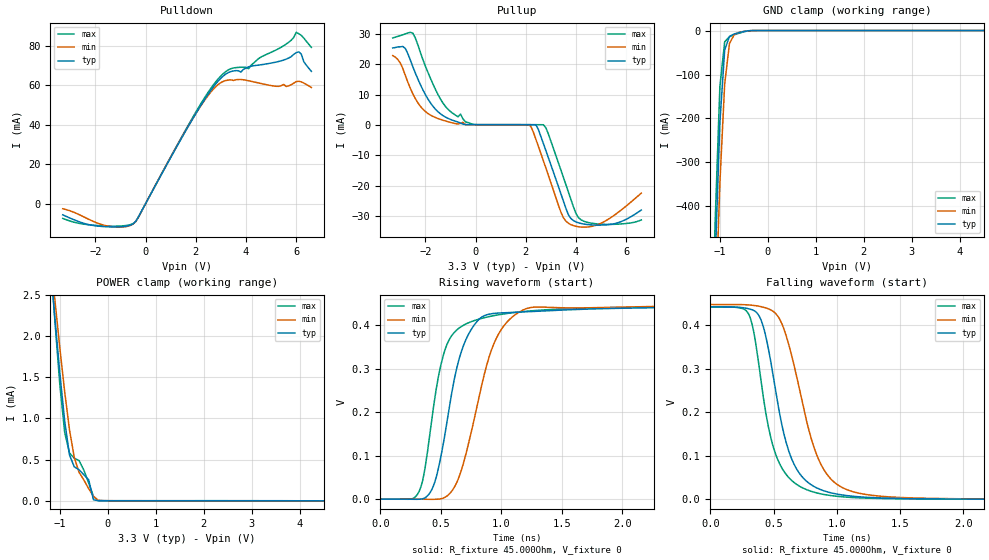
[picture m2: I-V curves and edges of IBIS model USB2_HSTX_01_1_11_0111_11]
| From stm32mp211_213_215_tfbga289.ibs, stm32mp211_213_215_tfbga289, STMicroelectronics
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[Model] USB2_HSTX_01_1_11_0111_11
Model_type   Output
Polarity   Non-Inverting
Enable   Active-High
C_comp   8.036pF   7.631pF   8.569pF
Vmeas = 200.000mV
Vref = 200.000mV
Rref = 45Ohms
Cref = 0pF
[Model Spec]
Vmeas   200.000mV   200.000mV   200.000mV
Vref   200.000mV   200.000mV   200.000mV
| This model is not intended for timing simulations.
| Warnings about Cref, Vref & Rref can be ignored
[Temperature Range]   25.000   125.000   -40.000
[Voltage Range]   3.300V   3.070V   3.630V
[GND Clamp Reference]   0.00V   0.00V   0.00V
[Pulldown Reference]   0.00V   0.00V   0.00V
[POWER Clamp Reference]   3.300V   3.070V   3.630V
[Pullup Reference]   3.300V   3.070V   3.630V
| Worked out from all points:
|   slope of the pulldown table from 0 to 0.495 V, typ, clamps not added: 42.6 ohm
|   GND clamp passes 1 mA (typ) near -0.43 V on its own axis
|   POWER clamp passes 1 mA (typ) near -0.91 V on its own axis
|   rising waveform, R_fixture 45.000Ohm, V_fixture 0: 20-80 % time 194ps typ, 246ps min, 169ps max; typ from 0 V to 0.442 V
|   falling waveform, R_fixture 45.000Ohm, V_fixture 0: 20-80 % time 196ps typ, 242ps min, 176ps max; typ from 0.442 V to 0 V
[GND Clamp]
-3.3V     -11.02A    -10.62A    -11.32A
-1.2V     -931.6mA   -1.049A    -855.7mA
-1.1V     -533.1mA   -671.7mA   -440.2mA
-1V       -209.4mA   -347mA     -127.3mA
-900mV    -44.44mA   -121.7mA   -25.6mA
-800mV    -13.15mA   -29.48mA   -14.15mA
-700mV    -7.742mA   -9.125mA   -9.769mA
-500mV    -2.127mA   -1.981mA   -2.893mA
-300mV    -19.47uA   -62.22uA   -13.66uA
6.6V      10.37uA    26.59uA    21.05uA
[Power Clamp]
-3.3V     3.206A     2.175A     4.855A
-1.2V     2.88mA     3.008mA    2.969mA
-1.1V     2.195mA    2.419mA    2.156mA
-1V       1.545mA    1.852mA    1.406mA
-900mV    967.6uA    1.324mA    831.4uA
-800mV    558uA      864.6uA    580.3uA
-700mV    412uA      525.9uA    517uA
-600mV    376.6uA    345uA      488.5uA
-400mV    254.2uA    146.6uA    216.8uA
-300mV    11.21uA    52.87uA    53.51uA
-100mV    94.85nA    985nA      361.1nA
6.6V      -2.75uA    -5.18uA    -3.448uA
[Pulldown]
-3.3V     -5.671mA   -2.581mA   -7.449mA
-1.6V     -11.64mA   -11.09mA   -11.31mA
-500mV    -10.25mA   -10.32mA   -10.1mA
1.9V      43.42mA    43.46mA    44.13mA
2.9V      62.15mA    60.37mA    63.26mA
3.4V      66.87mA    62.63mA    68.29mA
4.1V      69.19mA    62.19mA    68.26mA
4.5V      70.11mA    61.06mA    73.4mA
5.6V      73.12mA    59.29mA    80.76mA
6V        76.42mA    61.79mA    86.69mA
6.1V      76.81mA    61.93mA    85.99mA
6.6V      66.95mA    58.79mA    79.1mA
[Pullup]
-3.3V     25.37mA    22.87mA    28.68mA
-2.8V     25.24mA    16.38mA    30mA
-2.5V     19.22mA    10.28mA    30.28mA
-1.7V     6.185mA    2.83mA     13.54mA
-1.2V     2.603mA    1.31mA     6.112mA
-400mV    111.7uA    77.66uA    1.021mA
2.2V      68.59uA    -465uA     104.8uA
2.4V      56.18uA    -4.685mA   90.82uA
2.8V      -8.459mA   -14.22mA   -920uA
3.7V      -29.65mA   -32.41mA   -22.19mA
4.3V      -32.64mA   -33.68mA   -31.68mA
6.6V      -28.04mA   -22.46mA   -31.3mA
[Ramp]
R_load=45.000Ohm
dV/dt_r   633.016mV/985.000ps  601.227mV/995.000ps  686.729mV/930.000ps
dV/dt_f   635.188mV/225.000ps  604.117mV/285.000ps  688.534mV/210.000ps
[Rising waveform]
R_fixture=45.000Ohm
V_fixture=0
0s        452.3nV    3.134uV    468.1nV
320ps     -485.8uV   -405.8uV   17.12mV
370ps     3.021mV    -585.3uV   71.64mV
450ps     38.73mV    -570.3uV   231.4mV
590ps     243.5mV    18.02mV    376.2mV
720ps     374.6mV    117.3mV    404.9mV
920ps     426.8mV    344.2mV    421.4mV
1.07ns    429.5mV    414.2mV    428.3mV
1.28ns    432.2mV    442.1mV    434.2mV
9.9ns     442.5mV    448.1mV    442.6mV
[Falling waveform]
R_fixture=45.000Ohm
V_fixture=0
0s        441.9mV    447.5mV    442.1mV
310ps     437.2mV    446.4mV    421mV
420ps     395.5mV    441.3mV    232.6mV
530ps     225.9mV    422mV      93.32mV
680ps     70.6mV     285.1mV    34.73mV
810ps     31.07mV    127.6mV    17.17mV
930ps     16.64mV    54.26mV    9.574mV
1.16ns    6.152mV    15.02mV    3.583mV
1.71ns    1.121mV    2.357mV    826.5uV
9.9ns     14.45uV    30.67uV    5.121uV
